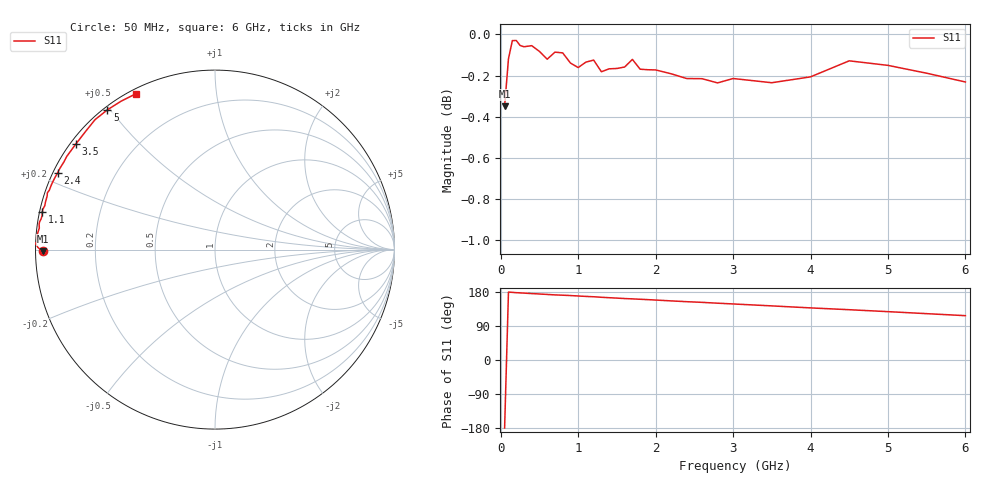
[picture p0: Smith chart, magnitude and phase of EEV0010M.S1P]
! Infineon Technologies  Discrete & RF Semiconductors
! BBY55-02W
! Si Tuning Diode in SCD-80
! VR =
! S-Parameters:  June  2000
# GHz  S  MA  R  50
!  f  S11
! GHz  MAG  ANG
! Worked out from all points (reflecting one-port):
!   34 points, 50 MHz to 6 GHz, reference 50 ohm
!   lowest |S11| = -0.3 dB at 50 MHz (marker M1), VSWR 49.76, Z = 1 - j0.262 ohm
!   phase of S11 starts at -179 deg and turns -64 deg over the sweep
!   S11 on the Smith chart (normalised r, x): 50 MHz: 0.02, -0.01; 1.1 GHz: 0.01, +0.11; 2.4 GHz: 0.01, +0.23; 3.5 GHz: 0.02, +0.34; 5 GHz: 0.01, +0.49; 6 GHz: 0.02, +0.61
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0.05  0.9606 -179.4
0.1  0.9865 179.3
0.15  0.9965 178.4
0.2  0.9966 177.7
0.25  0.9938 177.1
0.4  0.9937 175.3
0.6  0.9862 173.0
0.7  0.9901 171.8
0.8  0.9897 171.0
0.9  0.9841 170.1
1  0.9816 168.9
1.1  0.9846 167.8
1.2  0.9857 166.9
1.3  0.9793 165.5
1.6  0.9819 162.2
1.7  0.9861 161.3
1.8  0.9807 160.3
2  0.9803 158.2
2.4  0.9756 153.9
2.6  0.9755 152.1
2.8  0.9732 149.9
3  0.9756 147.9
3.5  0.9733 142.8
4  0.9765 137.5
4.5  0.9853 132.7
5  0.9828 127.6
5.5  0.9785 122.3
6  0.9737 117.0
